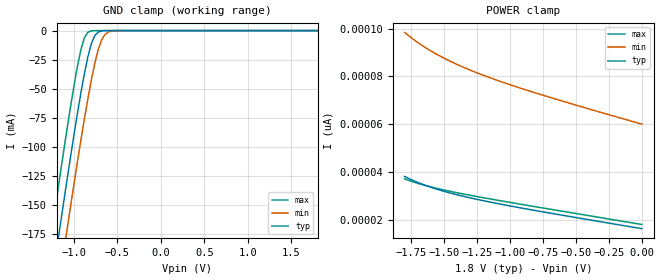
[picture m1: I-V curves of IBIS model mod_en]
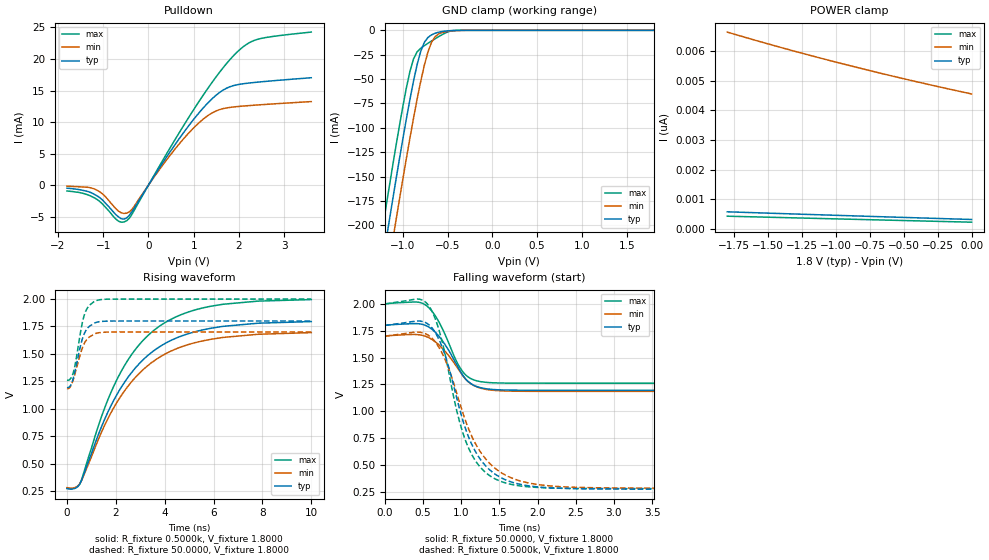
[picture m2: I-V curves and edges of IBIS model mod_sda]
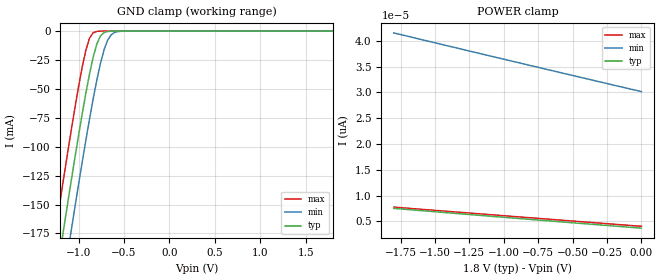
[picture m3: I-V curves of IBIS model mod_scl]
| IBIS (I/O, Buffer, Information, Specification) Model, officially
| electronic behavioral standard for Buffer structures of digital pins.
[IBIS ver]  4.0
[File name] m24c04_fa1_tssop8.ibs
[File Rev]  1.0
[Date]   11 June 2014
[Source]   CAD & Design Services (Catania) - STMicroelectronics
[Notes]
   (Note1)  This IBIS model includes the TSSOP8 package data
   (Note2)  This IBIS model has some Notes about the non-monotonicity
   of the I-V curves, but they are not indicative of problems
   inside the model;
[Copyright] (c) 2014 STMicroelectronics
|   Component M24C04
[Component] M24C04
[Manufacturer] STMicroelectronics
[Package]
| variable   typ   min   max
R_pkg   0.0   0.0   0.0
L_pkg   0.0H   0.0H   0.0H
C_pkg   0.0F   0.0F   0.0F
[Pin]  signal_name   model_name   R_pin   L_pin   C_pin
1   NC   NC   NA   NA   NA
2   E1   mod_en   NA   NA   NA
3   E2   mod_en   NA   NA   NA
4   VSS   GND   NA   NA   NA
5   SDA   mod_sda   NA   NA   NA
6   SCL   mod_scl   NA   NA   NA
7   WCN   mod_wc   NA   NA   NA
8   VCC   POWER   NA   NA   NA
[Package Model]  182696_TSSOP8
[Define Package Model]  182696_TSSOP8
[Manufacturer]  STMicroelectronics
[OEM]  STMicroelectronics
[Description]  8 pin TSSOP package
[Number Of Pins]  8
[Pin Numbers]
|Pin Num   Terminal Name
1   | net1
2   | net2
3   | net3
4   | net4_GND
5   | net5
6   | net6
7   | net7
8   | net8_VDD
[Model Data]
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[End Model Data]
[End Package Model]
| Models and submodels in the file (4): mod_en (Input), mod_sda (I/O_open_drain), mod_scl (Input), mod_wc (Input)
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|   Model mod_en
[Model]   mod_en
Model_type Input
Vinl   =   0.540V
Vinh   =   1.260V
C_comp   1.763pF   1.683pF   1.933pF
[Temperature Range]  25.0000   85.0000   -40.0000
[Voltage Range]   1.8000V   1.7000V   2.0000V
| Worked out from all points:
|   GND clamp passes 1 mA (typ) near -0.71 V on its own axis
[GND_clamp]
|Voltage   I(typ)   I(min)   I(max)
-1.8V     -506.7mA   -549.3mA   -463.8mA
-1.28V    -230.6mA   -274mA     -186.5mA
-1.24V    -209.8mA   -253.3mA   -165.8mA
-1.16V    -168.9mA   -212.2mA   -124.8mA
-1.08V    -128.7mA   -171.8mA   -85.14mA
-920mV    -53.64mA   -94.29mA   -16.44mA
-840mV    -22.68mA   -58.76mA   -1.468mA
-800mV    -11.31mA   -42.6mA    -261.9uA
-720mV    -1.249mA   -16.25mA   -6.98uA
-680mV    -318.6uA   -7.797mA   -1.128uA
-600mV    -18.77uA   -1.043mA   -29.45nA
1.8V      3.674pA    30.76pA    3.627pA
[POWER_clamp]
|Voltage   I(typ)   I(min)   I(max)
-1.8V     38.27pA    98.38pA    37.26pA
-1.74V    36.71pA    95.75pA    36.1pA
-1.68V    35.34pA    93.41pA    35.09pA
-1.56V    33.05pA    89.37pA    33.37pA
-1.42V    30.89pA    85.46pA    31.68pA
-1.24V    28.59pA    81.28pA    29.78pA
-1.04V    26.39pA    77.3pA     27.83pA
-800mV    23.99pA    73.02pA    25.58pA
-460mV    20.76pA    67.4pA     22.45pA
0V        16.5pA     60.1pA     18.24pA
|   Model mod_sda
[Model]   mod_sda
Model_type I/O_open_drain
Polarity   Non-Inverting
Vinl   =   0.540V
Vinh   =   1.260V
Vmeas  =   0.900V
Cref   =   10pF
Rref   =   1k
Vref   =   1.800V
C_comp   3.856pF   3.682pF   4.038pF
[Temperature Range]  25.0000   85.0000   -40.0000
[Voltage Range]   1.8000V   1.7000V   2.0000V
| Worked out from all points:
|   slope of the pulldown table from 0 to 0.27 V, typ, clamps not added: 89.1 ohm
|   GND clamp passes 1 mA (typ) near -0.55 V on its own axis
|   rising waveform, R_fixture 0.5000k, V_fixture 1.8000: 20-80 % time 2.36ns typ, 2.41ns min, 2.27ns max; typ from 0.272 V to 1.79 V
|   rising waveform, R_fixture 50.0000, V_fixture 1.8000: 20-80 % time 395ps typ, 423ps min, 367ps max; typ from 1.2 V to 1.8 V
|   falling waveform, R_fixture 50.0000, V_fixture 1.8000: 20-80 % time 310ps typ, 334ps min, 290ps max; typ from 1.8 V to 1.2 V
|   falling waveform, R_fixture 0.5000k, V_fixture 1.8000: 20-80 % time 424ps typ, 483ps min, 372ps max; typ from 1.8 V to 0.272 V
[Pulldown]
|Voltage   I(typ)   I(min)   I(max)
-1.8V     -476.6uA   -158uA     -917.6uA
-1.2V     -1.433mA   -578uA     -1.982mA
-1.02V    -2.311mA   -1.342mA   -2.943mA
-660mV    -5.033mA   -4.116mA   -5.712mA
-480mV    -5.187mA   -4.43mA    -5.63mA
-360mV    -4.148mA   -3.803mA   -4.555mA
420mV     4.66mA     4.177mA    5.2mA
1.02V     10.61mA    9.227mA    12.19mA
1.5V      14.28mA    11.78mA    17.2mA
1.92V     15.85mA    12.43mA    20.81mA
2.4V      16.32mA    12.71mA    23.09mA
3.6V      17.03mA    13.25mA    24.26mA
[GND_clamp]
|Voltage   I(typ)   I(min)   I(max)
-1.8V     -578.3mA   -619mA     -545mA
-1.24V    -246.2mA   -288.1mA   -211.3mA
-1.2V     -223.1mA   -265.1mA   -188.2mA
-1.16V    -200.3mA   -242.2mA   -165.3mA
-1.08V    -155.2mA   -197mA     -120.6mA
-960mV    -90.68mA   -131.3mA   -58.9mA
-880mV    -51.81mA   -89.93mA   -29.19mA
-800mV    -21.5mA    -52.3mA    -18.39mA
-680mV    -4.704mA   -12.46mA   -10.99mA
-600mV    -1.891mA   -3.59mA    -6.485mA
-400mV    -80.51uA   -346.4uA   -50.5uA
1.8V      316.9pA    4.657nA    202.8pA
[POWER_clamp]
|Voltage   I(typ)   I(min)   I(max)
-1.8V     576.3pA    6.648nA    427.7pA
-1.38V    513.5pA    6.097nA    380.4pA
-940mV    449.3pA    5.564nA    330.9pA
-500mV    386.6pA    5.072nA    281.4pA
0V        316.9pA    4.558nA    225.3pA
[Ramp]
| variable   typ   min   max
dV/dt_r   0.3632/0.4912n   0.3093/0.5282n   0.4437/0.4398n
dV/dt_f   0.3632/0.3649n   0.3093/0.3824n   0.4437/0.3452n
R_load = 50.0000
[Rising Waveform]
R_fixture= 0.5000k
V_fixture= 1.8000
V_fixture_min= 1.7000
V_fixture_max= 2.0000
|time   V(typ)   V(min)   V(max)
0s        272.2mV    280.9mV    276.5mV
320ps     274mV      281.2mV    278.4mV
520ps     311.6mV    315.2mV    312.8mV
1.42ns    840.1mV    790.2mV    932.7mV
2ns       1.112V     1.042V     1.246V
2.72ns    1.351V     1.266V     1.517V
3.56ns    1.53V      1.436V     1.715V
4.64ns    1.659V     1.561V     1.855V
5.88ns    1.733V     1.633V     1.934V
10ns      1.795V     1.694V     1.995V
[Rising Waveform]
R_fixture= 50.0000
V_fixture= 1.8000
V_fixture_min= 1.7000
V_fixture_max= 2.0000
|time   V(typ)   V(min)   V(max)
0s        1.195V     1.184V     1.261V
140ps     1.211V     1.201V     1.274V
260ps     1.28V      1.266V     1.331V
360ps     1.374V     1.344V     1.434V
600ps     1.614V     1.535V     1.755V
740ps     1.7V       1.608V     1.874V
900ps     1.748V     1.651V     1.938V
1.22ns    1.789V     1.689V     1.987V
1.94ns    1.8V       1.7V       2V
10ns      1.8V       1.7V       2V
[Falling Waveform]
R_fixture= 50.0000
V_fixture= 1.8000
V_fixture_min= 1.7000
V_fixture_max= 2.0000
|time   V(typ)   V(min)   V(max)
0s        1.8V       1.7V       2V
400ps     1.816V     1.715V     2.018V
550ps     1.794V     1.693V     1.981V
650ps     1.743V     1.652V     1.899V
750ps     1.66V      1.588V     1.773V
930ps     1.446V     1.425V     1.476V
1.03ns    1.325V     1.322V     1.359V
1.15ns    1.247V     1.245V     1.295V
1.31ns    1.21V      1.205V     1.27V
10ns      1.195V     1.184V     1.261V
[Falling Waveform]
R_fixture= 0.5000k
V_fixture= 1.8000
V_fixture_min= 1.7000
V_fixture_max= 2.0000
|time   V(typ)   V(min)   V(max)
0s        1.8V       1.7V       2V
440ps     1.841V     1.737V     2.045V
580ps     1.803V     1.702V     1.977V
780ps     1.539V     1.495V     1.558V
960ps     1.069V     1.123V     950.4mV
1.1ns     751.9mV    827.6mV    649.4mV
1.32ns    489.3mV    554.1mV    427.3mV
1.62ns    348mV      388.9mV    322.5mV
2.64ns    275.4mV    286.9mV    278.3mV
10ns      272.2mV    280.9mV    276.5mV
|   Model mod_scl
[Model]   mod_scl
Model_type Input
Vinl   =   0.540V
Vinh   =   1.260V
C_comp   1.763pF   1.683pF   1.933pF
[Temperature Range]  25.0000   85.0000   -40.0000
[Voltage Range]   1.8000V   1.7000V   2.0000V
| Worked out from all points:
|   GND clamp passes 1 mA (typ) near -0.71 V on its own axis
[GND_clamp]
|Voltage   I(typ)   I(min)   I(max)
-1.8V     -506.7mA   -549.3mA   -463.8mA
-1.28V    -230.6mA   -274mA     -186.5mA
-1.24V    -209.8mA   -253.3mA   -165.8mA
-1.16V    -168.9mA   -212.2mA   -124.8mA
-1.08V    -128.7mA   -171.8mA   -85.14mA
-920mV    -53.64mA   -94.29mA   -16.44mA
-840mV    -22.68mA   -58.76mA   -1.468mA
-800mV    -11.31mA   -42.6mA    -261.9uA
-720mV    -1.249mA   -16.25mA   -6.98uA
-680mV    -318.6uA   -7.797mA   -1.128uA
-600mV    -18.77uA   -1.043mA   -29.45nA
1.8V      3.674pA    30.76pA    3.627pA
[POWER_clamp]
|Voltage   I(typ)   I(min)   I(max)
-1.8V     7.509pA    41.51pA    7.748pA
-940mV    5.652pA    36.04pA    5.962pA
-440mV    4.594pA    32.89pA    4.934pA
0V        3.674pA    30.14pA    4.034pA
